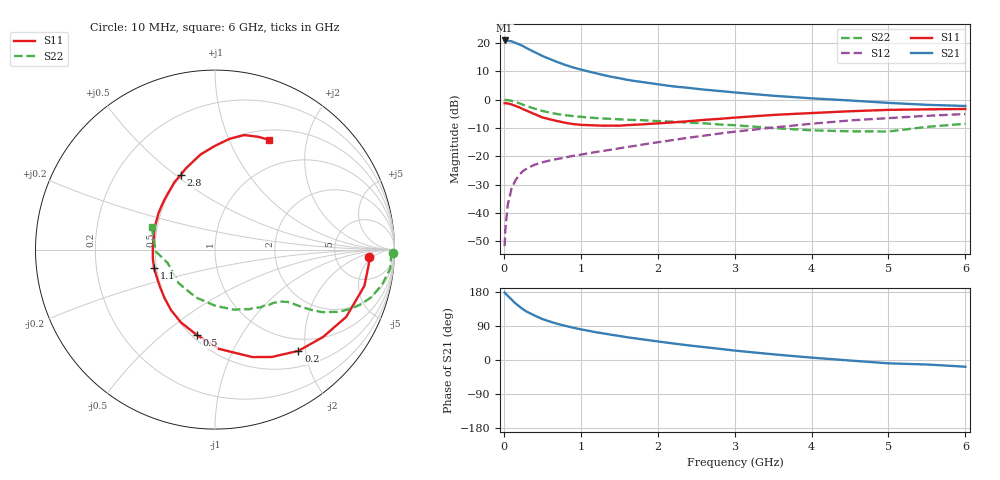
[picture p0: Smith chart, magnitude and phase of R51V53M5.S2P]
! SIEMENS Small Signal Semiconductors
! BFR183
! Si NPN RF Bipolar Junction Transistor in SOT23
! VCE = 1.5 V  IC = 3.5 mA
! Common Emitter S-Parameters:  May  1996
# GHz  S  MA  R  50
!  f  S11  S21  S12  S22
! GHz  MAG  ANG  MAG  ANG  MAG  ANG  MAG  ANG
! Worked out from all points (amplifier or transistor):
!   36 points, 10 MHz to 6 GHz, reference 50 ohm
!   highest |S21| = 20.9 dB at 10 MHz (marker M1)
!   |S21| within 3 dB of that: start of sweep to 317.3 MHz
!   unconditionally stable (mu >= 1): 1.167 GHz to 2.78 GHz
!   at 250 MHz: K = 0.33, MSG = 22.0 dB, |S12| = -25.2 dB
!   at 1.4 GHz: K = 1.07, MAG = 11.3 dB, |S12| = -17.7 dB
!   at 6 GHz: K = 0.91, MSG = 1.4 dB, |S12| = -5.1 dB
!   S11 on the Smith chart (normalised r, x): 10 MHz: 12, -4; 200 MHz: 0.77, -1.87; 500 MHz: 0.53, -0.66; 1.1 GHz: 0.48, -0.11; 2.8 GHz: 0.50, +0.52; 6 GHz: 0.62, +1.42
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0.01  0.8602 -2.9  11.03 178.1  0.0026 85.6  0.9939 -1.2
0.02  0.8608 -5.5  10.92 175.7  0.0052 89.9  0.9816 -2.4
0.05  0.8565 -13.7  10.89 169.6  0.0137 82.0  0.9826 -6.1
0.1  0.8218 -27.1  10.69 159.6  0.0269 76.2  0.9506 -11.9
0.15  0.7741 -39.0  9.968 149.7  0.0374 70.1  0.9106 -16.9
0.2  0.731 -50.5  9.437 141.4  0.0469 64.8  0.864 -20.9
0.25  0.6773 -62.0  8.764 133.7  0.0549 60.5  0.811 -24.4
0.3  0.6341 -70.8  8.023 127.4  0.061 57.5  0.7664 -26.9
0.4  0.5534 -87.8  6.862 117.3  0.071 53.1  0.6927 -30.2
0.5  0.4858 -102.2  5.895 108.1  0.0782 50.7  0.6317 -32.1
0.6  0.4477 -115.2  5.17 101.3  0.0845 49.6  0.587 -33.3
0.7  0.4166 -126.1  4.574 95.3  0.0899 49.3  0.5547 -34.1
0.9  0.3707 -145.6  3.688 85.3  0.1017 49.4  0.5116 -35.3
1.1  0.3545 -163.6  3.133 77.1  0.1129 50.8  0.4835 -37.0
1.4  0.3473 174.8  2.518 66.6  0.131 52.7  0.4564 -39.9
1.6  0.3543 163.1  2.238 60.1  0.1455 53.4  0.441 -42.3
2.2  0.3958 135.5  1.71 43.7  0.1935 53.7  0.4087 -52.0
2.8  0.4571 114.7  1.419 29.6  0.2514 50.8  0.3641 -65.6
3.5  0.5359 98.7  1.169 15.0  0.321 44.2  0.3143 -89.1
4.5  0.6227 82.5  0.964 -1.4  0.4294 31.9  0.2757 -137.6
5.5  0.6727 69.1  0.809 -11.9  0.5176 18.9  0.3304 -178.2
6  0.6824 63.8  0.771 -17.7  0.5563 10.4  0.3745 160.3
